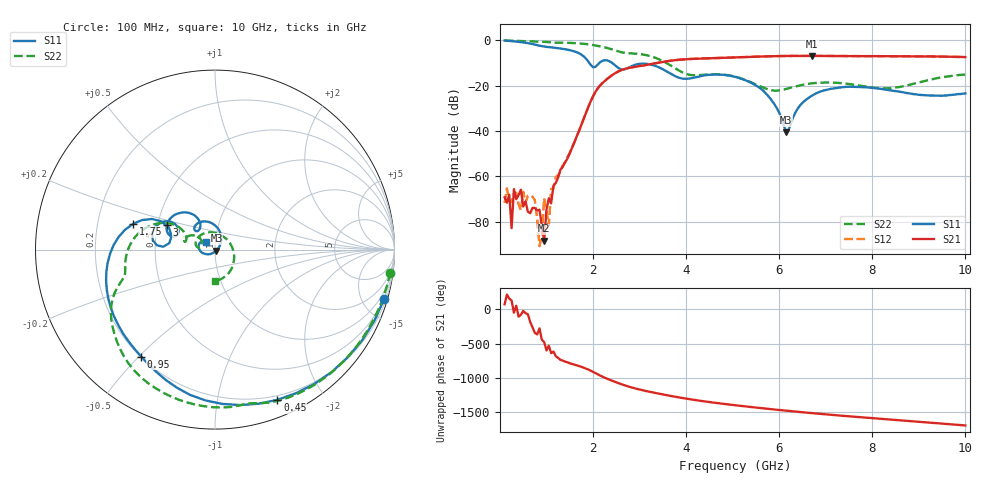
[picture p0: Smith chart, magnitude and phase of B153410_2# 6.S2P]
!  2-Port S-parameters saved by WinCal
! VAR MeasName=S-Parameters (CALIBRATED_DATA) read from VNA (N5245A)
! VAR MeasDate=2016-12-23 9:59:39
! VAR NAME=B153410_2# 6
! VAR FILENAME=B153410_2# 6.S2P
! VAR DATE=2016-12-23 9:59:39
! VAR PHYS_PORTS=1,2
# Hz S DB R 50
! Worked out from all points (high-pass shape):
!   199 points, 100 MHz to 10 GHz, reference 50 ohm
!   highest |S21| = -6.93 dB at 6.7 GHz (marker M1); lowest = -88.3 dB at 950 MHz (marker M2)
!   |S21| within 3 dB of the highest: 3.406 GHz to end of sweep
!   lowest |S11| = -40.6 dB at 6.15 GHz (marker M3), VSWR 1.02, Z = 50.8 - j0.522 ohm
!   |S11| at or under -10 dB: 1.919 GHz to 2.138 GHz (219.5 MHz wide, 10.8 % of centre); 2.408 GHz to end of sweep
!   |S22| runs from -22.2 to -0.1 dB; largest |S21 - S12| = 0.0023
!   S11 on the Smith chart (normalised r, x): 100 MHz: 0.45, -7.01; 450 MHz: 0.16, -1.49; 950 MHz: 0.20, -0.51; 1.75 GHz: 0.36, +0.13; 3 GHz: 0.56, +0.17; 10 GHz: 0.90, +0.08
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1e8  -0.16 -16.2  -69.26 74.4  -71.70 111.1  -0.13 -7.5
2e8  -0.32 -31.5  -68.09 157.6  -70.79 103.5  -0.21 -14.3
2.5e8  -0.42 -39.0  -82.81 128.8  -71.33 112.3  -0.24 -17.7
3e8  -0.51 -46.3  -65.61 -48.8  -67.62 -57.6  -0.28 -21.0
4.5e8  -0.86 -67.5  -65.88 -80.6  -74.99 -96.6  -0.36 -30.9
5e8  -0.99 -74.2  -73.32 -22.7  -66.81 -92.7  -0.40 -34.2
6.5e8  -1.50 -93.7  -76.25 175.0  -68.31 40.1  -0.48 -44.1
9e8  -2.63 -120.2  -81.93 -84.7  -85.75 -6.2  -0.67 -60.5
9.5e8  -2.80 -124.6  -88.33 -119.3  -69.62 -170.4  -0.73 -63.8
1.05e9  -3.07 -133.3  -69.64 -173.2  -81.55 77.3  -0.87 -70.3
1.1e9  -3.18 -137.6  -71.91 79.3  -65.59 112.1  -0.98 -73.4
1.75e9  -6.39 162.6  -37.25 -121.6  -37.21 -122.1  -1.52 -113.5
2.2e9  -9.11 171.4  -18.94 95.1  -18.93 94.9  -2.92 -143.0
3e9  -10.43 153.2  -11.42 -94.1  -11.41 -94.2  -6.11 -176.4
3.4e9  -11.84 126.4  -9.95 -152.6  -9.94 -152.6  -8.27 160.0
4.25e9  -16.15 136.2  -8.15 106.4  -8.15 106.3  -15.46 163.8
5.05e9  -16.16 101.4  -7.58 36.2  -7.60 36.3  -16.07 149.8
5.75e9  -24.27 54.3  -7.13 -16.1  -7.14 -16.0  -21.60 151.1
6.15e9  -40.55 -33.2  -6.96 -43.7  -6.96 -43.7  -21.50 170.5
6.7e9  -24.49 -155.9  -6.93 -79.3  -6.93 -79.4  -19.04 164.6
8.35e9  -22.00 142.4  -7.08 -172.9  -7.06 -172.9  -21.20 41.9
1e10  -23.47 140.7  -7.46 100.1  -7.48 100.1  -15.14 -89.7
